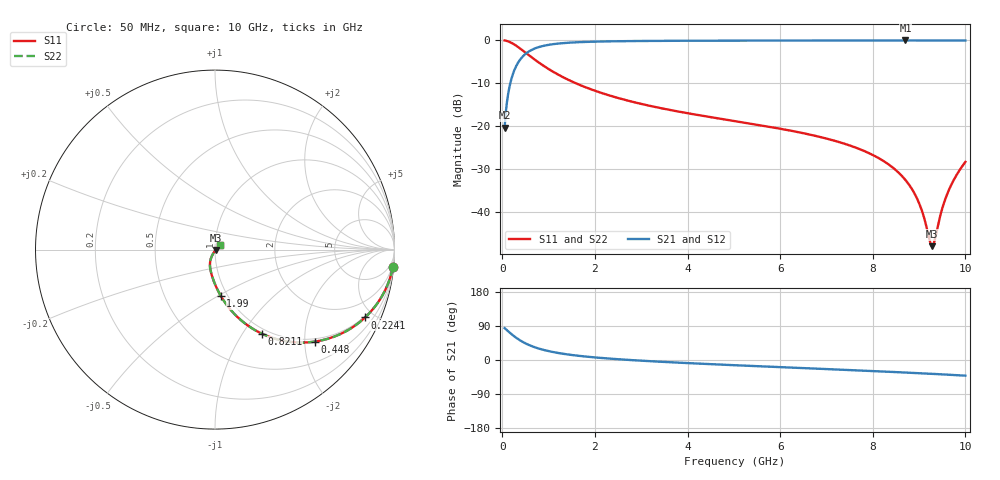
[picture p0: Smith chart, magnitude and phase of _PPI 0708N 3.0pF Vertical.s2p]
! S-Parameter data specifications (vertical orientation):
! Substrate: 40-mil Rogers 3003C, Substrate thickness, H=1.016mm, Dielectric constant, Er=3, Conductor thickness, T_mtl=0.043mm, Loss Tangent, Tand=0.003
! PCB Mounting Pad Footprint: Pad width, PadW=2.54mm , Pad length, PadL=0.51mm , Pad gap, PadG (edge-to-edge)=0.71mm , Reference planes=1.73mm apart
! Created Tue Jan 16 08:44:54 2018
# GHz S MA R 50
! 2 Port Network Data from SP1.SP block
! freq  magS11  angS11  magS21  angS21  magS12  angS12  magS22  angS22
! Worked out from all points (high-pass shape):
!   801 points, 50 MHz to 10 GHz, reference 50 ohm
!   highest |S21| = -0.04 dB at 8.707 GHz (marker M1); lowest = -20.3 dB at 50 MHz (marker M2)
!   |S21| within 3 dB of the highest: 516.5 MHz to end of sweep
!   lowest |S11| = -47.9 dB at 9.279 GHz (marker M3), VSWR 1.01, Z = 50.3 - j0.262 ohm
!   |S11| at or under -10 dB: 1.588 GHz to end of sweep
!   |S22| runs from -47.9 to 0.0 dB; largest |S21 - S12| = 0
!   S11 on the Smith chart (normalised r, x): 50 MHz: 1, -20; 224.1 MHz: 0.93, -4.46; 448 MHz: 0.93, -2.23; 821.1 MHz: 0.93, -1.22; 1.99 GHz: 0.93, -0.51; 10 GHz: 1.06, +0.05
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0.05  0.9954 -5.7  0.09613 84.3  0.09613 84.3  0.9954 -5.7
0.1370625  0.9667 -15.4  0.2559 74.6  0.2559 74.6  0.9667 -15.4
0.224125  0.9177 -24.3  0.3971 65.7  0.3971 65.7  0.9177 -24.3
0.448  0.7566 -42.6  0.6535 47.3  0.6535 47.3  0.7566 -42.6
0.821125  0.5355 -60.9  0.8439 29.0  0.8439 29.0  0.5355 -60.9
1.19425  0.4019 -71.1  0.9148 18.8  0.9148 18.8  0.4019 -71.1
1.716625  0.2956 -79.7  0.9542 10.1  0.9542 10.1  0.2956 -79.7
1.99025  0.2599 -82.9  0.9645 6.9  0.9645 6.9  0.2599 -82.9
3.370812  0.1643 -93.8  0.9848 -4.3  0.9848 -4.3  0.1643 -93.8
5.025  0.1146 -102.9  0.9914 -13.8  0.9914 -13.8  0.1146 -102.9
6.691625  0.07868 -110.6  0.9943 -22.4  0.9943 -22.4  0.07868 -110.6
7.674188  0.05518 -114.6  0.9954 -27.4  0.9954 -27.4  0.05518 -114.6
8.345812  0.03574 -116.0  0.9958 -31.1  0.9958 -31.1  0.03574 -116.0
8.7065  0.02358 -114.7  0.9959 -33.1  0.9959 -33.1  0.02358 -114.7
8.992563  0.01298 -108.2  0.9959 -34.8  0.9959 -34.8  0.01298 -108.2
9.1045  0.008721 -99.6  0.9958 -35.5  0.9958 -35.5  0.008721 -99.6
9.228875  0.004665 -68.6  0.9957 -36.2  0.9957 -36.2  0.004665 -68.6
9.278625  0.004005 -40.6  0.9956 -36.5  0.9956 -36.5  0.004005 -40.6
9.328375  0.00451 -10.8  0.9956 -36.8  0.9956 -36.8  0.00451 -10.8
9.490063  0.01056 28.4  0.9953 -37.9  0.9953 -37.9  0.01056 28.4
9.626875  0.0172 36.3  0.995 -38.7  0.995 -38.7  0.0172 36.3
10  0.03836 41.1  0.9938 -41.3  0.9938 -41.3  0.03836 41.1
